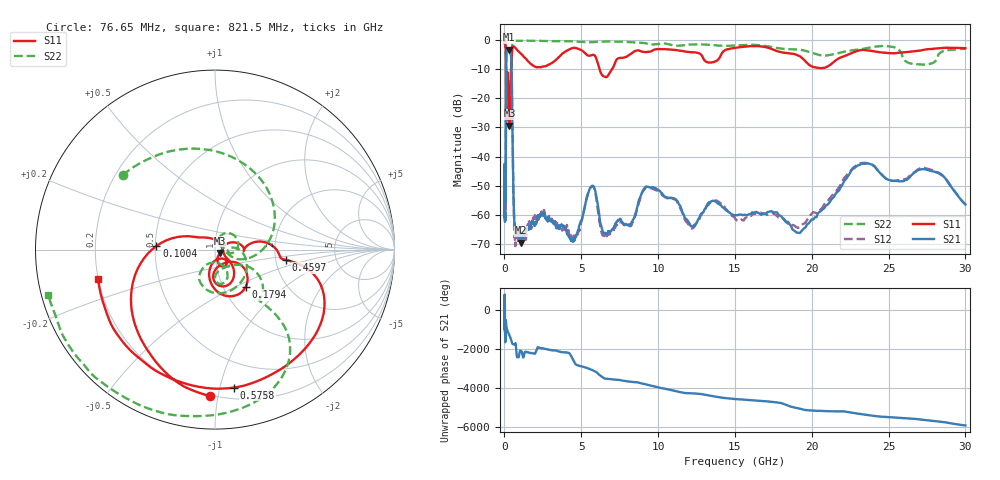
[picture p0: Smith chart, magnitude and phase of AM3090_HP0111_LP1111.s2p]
! Date/Time: Thu, Feb 28, 2019 2:01 PM
! Network Analyzer: Agilent Technologies E8364B Rev: A.07.50.67
! Sweep from 0.010 to 30.000 GHz, 1601 Points, Sweep Type: LOG
! Power Supply: 5.023 V, 0.002 A
# Hz S DB R 50
!freq MagS11 AngS11 MagS21 AngS21 MagS12 AngS12 MagS22 AngS22
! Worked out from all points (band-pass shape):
!   1601 points, 10 MHz to 30 GHz, reference 50 ohm
!   highest |S21| = -3.37 dB at 270.5 MHz (marker M1); lowest = -69.4 dB at 1.05 GHz (marker M2)
!   |S21| within 3 dB of the highest: 117.3 MHz to 442.1 MHz (324.8 MHz wide, 116 % of centre)
!   lowest |S11| = -29.4 dB at 323.9 MHz (marker M3), VSWR 1.07, Z = 52.9 - j1.93 ohm
!   |S11| at or under -10 dB: 100.6 MHz to 430.4 MHz (329.7 MHz wide, 124 % of centre); 6.184 GHz to 7.011 GHz (827.5 MHz wide, 12.5 % of centre)
!   |S22| runs from -28.2 to -0.2 dB; largest |S21 - S12| = 0.012
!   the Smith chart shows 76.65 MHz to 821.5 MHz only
!   S11 on the Smith chart (normalised r, x): 76.65 MHz: 0.19, -0.95; 100.4 MHz: 0.51, +0.02; 179.4 MHz: 1.27, -0.57; 459.7 MHz: 2.29, -0.31; 575.8 MHz: 0.29, -1.11; 821.5 MHz: 0.20, -0.12
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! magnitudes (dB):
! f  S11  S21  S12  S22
! 10 MHz  -0.3  -44.2  -43.5  -0.7
! 38.04 MHz  -0.5  -60.4  -59.7  -1.7
! 76.65 MHz  -1.8  -54.2  -54.9  -3.6
! 100.4 MHz  -9.7  -19.9  -19.9  -10.7
! 109.3 MHz  -27.8  -9.0  -9.0  -27.5
! 144.7 MHz  -20.5  -4.2  -4.1  -22.2
! 179.4 MHz  -11.4  -3.7  -3.6  -13.7
! 270.5 MHz  -20.6  -3.4  -3.3  -18.8
! 323.9 MHz  -29.4  -3.5  -3.5  -19.3
! 459.7 MHz  -7.9  -8.5  -8.4  -7.7
! 550.5 MHz  -2.3  -42.7  -42.5  -0.5
! 575.8 MHz  -2.2  -50.5  -50.5  -0.4
! 821.5 MHz  -3.5  -65.0  -65.0  -0.3
! 1.05 GHz  -4.6  -69.4  -66.4  -0.3
! 2.084 GHz  -9.4  -62.8  -60.8  -0.3
! 4.458 GHz  -2.8  -69.0  -67.3  -0.5
! 5.697 GHz  -5.2  -50.2  -50.0  -0.8
! 7.926 GHz  -5.8  -63.1  -63.0  -0.7
! 9.49 GHz  -4.0  -50.6  -50.7  -1.6
! 19.31 GHz  -6.0  -65.6  -63.6  -3.4
! 23.36 GHz  -3.5  -42.4  -42.1  -3.1
! 30 GHz  -2.9  -56.4  -56.4  -3.1
